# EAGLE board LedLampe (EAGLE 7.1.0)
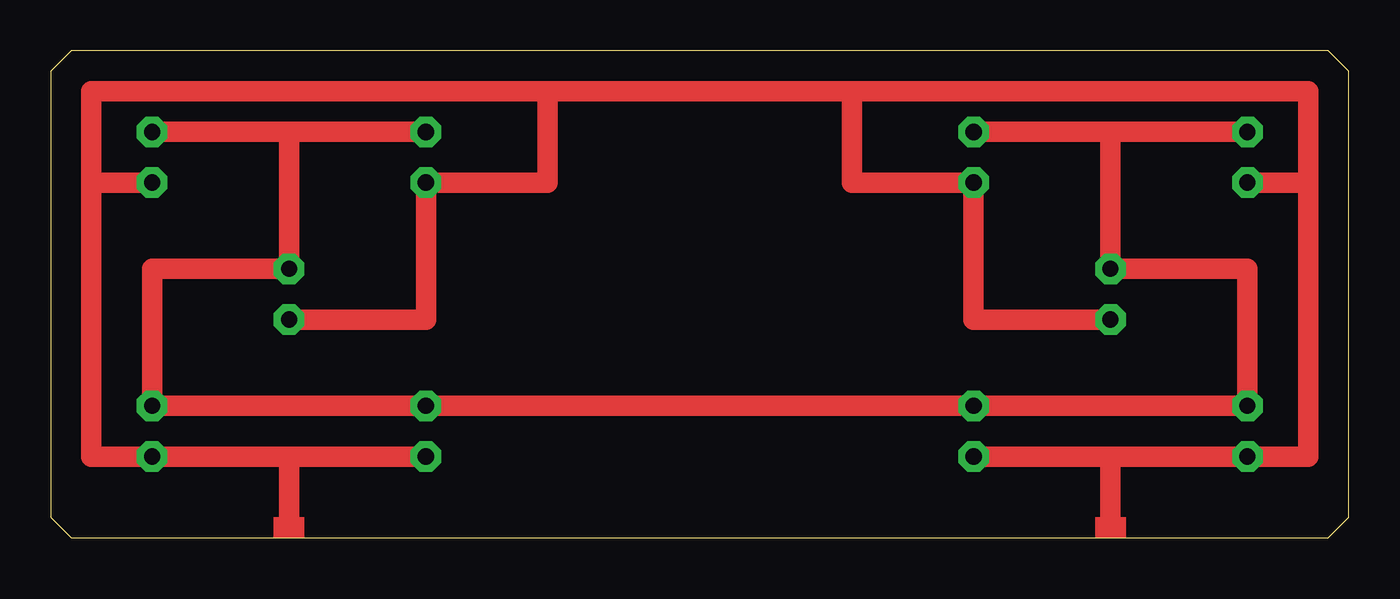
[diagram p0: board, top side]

Size 64 x 24 mm. Coordinates in mm from the lower left corner, seen from the top.
Outline: 0,1 1,0 63,0 64,1 64,23 63,24 1,24 0,23 0,1
Copper layers (1*16): Top 0.035mm / dielectric 1.5mm / Bottom 0.035mm
Design rules "default": minimum track width 10mil, minimum drill 24mil, track to track 8mil, track to pad 8mil, pad to pad 8mil, via to via 8mil, smd to smd 8mil, copper to edge 40mil, drill to drill 8mil, minimum pad ring 10mil, minimum via ring 8mil, stop-mask expansion 4mil, vias tented up to drill 0mil, thermal gap 10mil

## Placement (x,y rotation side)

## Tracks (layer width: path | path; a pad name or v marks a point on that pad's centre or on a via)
A  (via drill 0.8 pad 1.5)
  Top 1: 2,17.5 2,4 v5,4 11.75,4 | v5,17.5 2,17.5 | 2,17.5 2,22 24.5,22 | 24.5,22 24.5,17.5 v18.5,17.5 18.5,10.75 v11.75,10.75 | 11.75,4 v18.5,4 | 62,17.5 62,4 v59,4 52.25,4 | v59,17.5 62,17.5 | 62,17.5 62,22 39.5,22 | 39.5,22 39.5,17.5 v45.5,17.5 45.5,10.75 v52.25,10.75 | 52.25,4 v45.5,4 | 24.5,22 39.5,22 | 11.75,4 11.75,0.5 | 52.25,4 52.25,0.5
B  (via drill 0.8 pad 1.5)
  Top 1: v5,20 v18.5,20 11.75,20 v11.75,13.25 5,13.25 v5,6.5 v18.5,6.5 v45.5,6.5 v59,6.5 59,13.25 v52.25,13.25 52.25,20 | v59,20 52.25,20 | v45.5,20 52.25,20
(copper drawn outside any net)
  shapes: Top area x2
